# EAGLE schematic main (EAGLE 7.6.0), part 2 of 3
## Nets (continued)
U_DMA_9: IC37.15(D4)
U_DMA_10: IC38.15(D4)
U_DMA_11: IC40.15(D4)
U_DMA_12: IC41.15(D4)
U_DMA_13: IC71.15(D4)
U_DMA_14: IC20.15(D4)
U_DMA_15: IC172.15(D4)
U_FETCH_0: IC186.2(D2)
U_FETCH_1: IC160.2(D2)
U_FETCH_2: IC159.2(D2)
U_FETCH_3: IC142.2(D2)
U_FETCH_4: IC129.2(D2)
U_FETCH_5: IC73.2(D2)
U_FETCH_6: IC34.2(D2)
U_FETCH_7: IC35.2(D2)
U_FETCH_8: IC36.2(D2)
U_FETCH_9: IC37.2(D2)
U_FETCH_10: IC38.2(D2)
U_FETCH_11: IC40.2(D2)
U_FETCH_12: IC41.2(D2)
U_FETCH_13: IC71.2(D2)
U_FETCH_14: IC20.2(D2)
U_FETCH_15: IC172.2(D2)
U_FLAGS_REG_WRT: IC126.1(G)
U_INT_0: IC186.14(D5)
U_INT_1: IC160.14(D5)
U_INT_2: IC159.14(D5)
U_INT_3: IC142.14(D5)
U_INT_4: IC129.14(D5)
U_INT_5: IC73.14(D5)
U_INT_6: IC34.14(D5)
U_INT_7: IC35.14(D5)
U_INT_8: IC36.14(D5)
U_INT_9: IC37.14(D5)
U_INT_10: IC38.14(D5)
U_INT_11: IC40.14(D5)
U_INT_12: IC41.14(D5)
U_INT_13: IC71.14(D5)
U_INT_14: IC20.14(D5)
U_INT_15: IC172.14(D5)
U_OF: IC126.9(4Q) IC156.11(2C1)
U_OFFSET0: IC49.3(1B)
U_OFFSET1: IC49.6(2B)
U_OFFSET2: IC49.10(3B)
U_OFFSET3: IC49.13(4B)
U_OFFSET4: IC55.3(1B)
U_OFFSET5: IC55.6(2B)
U_OFFSET6: IC55.10(3B) IC55.13(4B) IC63.3(1B) IC63.6(2B) IC63.10(3B) IC63.13(4B) IC68.3(1B) IC68.6(2B) IC68.10(3B) IC68.13(4B)
U_SF: IC126.6(3Q) IC156.5(1C1)
U_TRAP_0: IC186.1(D3)
U_TRAP_1: IC160.1(D3)
U_TRAP_2: IC159.1(D3)
U_TRAP_3: IC142.1(D3)
U_TRAP_4: IC129.1(D3)
U_TRAP_5: IC73.1(D3)
U_TRAP_6: IC34.1(D3)
U_TRAP_7: IC35.1(D3)
U_TRAP_8: IC36.1(D3)
U_TRAP_9: IC37.1(D3)
U_TRAP_10: IC38.1(D3)
U_TRAP_11: IC40.1(D3)
U_TRAP_12: IC41.1(D3)
U_TRAP_13: IC71.1(D3)
U_TRAP_14: IC20.1(D3)
U_TRAP_15: IC172.1(D3)
U_ZF: IC46.1(A:I0) IC126.2(1Q) IC127.2(A:I1) IC155.5(1C1)
U_ZF_IN_SRC: IC121.1(!A!/B)
VAR_SPEED_CLK: SW1.4
VCC: IC8.2(A:D) IC8.4(A:PRE) IC39.2(A:D) IC39.4(A:PRE) IC49.2(1A) IC56.5(1C1) IC163.2(A:D) IC163.4(A:PRE) IC164.2(A:D) IC164.4(A:PRE) IC168.2(A:D) IC168.4(A:PRE) IC174.2(A:D) IC174.4(A:PRE) IC187.2(A:D) IC187.4(A:PRE) IC188.2(A:D) IC188.4(A:PRE) IC204.4(A:PRE) IC221.2(A:D) IC221.4(A:PRE) IC222.6(G1) IC413.1(A:CLR) R23.2 R24.2 R25.2 R26.2 RN7.9 RN7.10 RN7.11 RN7.12 RN7.13 RN7.14 RN7.15 RN7.16
WR: IC60.5(Q2) IC69.13(B:A2)
XBUS0: IC2.18(Y1) IC9.18(Y1) IC25.9(B:Y1) IC27.9(B:Y1) IC29.18(Y1) IC87.18(Y1) IC91.18(Y1) IC92.18(Y1) IC116.18(Y1) IC117.18(Y1) IC122.18(Y1) IC125.18(Y1) IC140.18(Y1) IC145.18(Y1) IC154.18(Y1) IC181.18(A:Y1) IC210.18(Y1) IC245.18(Y1)
XBUS1: IC2.17(Y2) IC9.17(Y2) IC25.7(B:Y2) IC27.7(B:Y2) IC29.17(Y2) IC87.17(Y2) IC116.17(Y2) IC117.17(Y2) IC122.17(Y2) IC125.17(Y2) IC145.17(Y2) IC154.17(Y2) IC181.16(A:Y2) IC245.17(Y2)
XBUS2: IC2.16(Y3) IC9.16(Y3) IC25.5(B:Y3) IC27.5(B:Y3) IC29.16(Y3) IC87.16(Y3) IC116.16(Y3) IC117.16(Y3) IC122.16(Y3) IC125.16(Y3) IC145.16(Y3) IC154.16(Y3) IC181.14(A:Y3) IC245.16(Y3)
XBUS3: IC2.15(Y4) IC9.15(Y4) IC25.3(B:Y4) IC27.3(B:Y4) IC29.15(Y4) IC87.15(Y4) IC116.15(Y4) IC117.15(Y4) IC122.15(Y4) IC125.15(Y4) IC145.15(Y4) IC154.15(Y4) IC181.12(A:Y4) IC245.15(Y4)
XBUS4: IC24.9(B:Y1) IC26.9(B:Y1) IC29.14(Y5) IC87.14(Y5) IC116.14(Y5) IC125.14(Y5) IC154.14(Y5) IC176.18(A:Y1) IC245.14(Y5)
XBUS5: IC24.7(B:Y2) IC26.7(B:Y2) IC29.13(Y6) IC87.13(Y6) IC116.13(Y6) IC125.13(Y6) IC154.13(Y6) IC176.16(A:Y2) IC245.13(Y6)
XBUS6: IC24.5(B:Y3) IC26.5(B:Y3) IC29.12(Y7) IC87.12(Y7) IC115.12(Y7) IC116.12(Y7) IC125.12(Y7) IC154.12(Y7) IC176.14(A:Y3) IC245.12(Y7)
XBUS7: IC2.11(Y8) IC3.11(Y8) IC9.11(Y8) IC24.3(B:Y4) IC26.3(B:Y4) IC29.11(Y8) IC80.4(B:I0) IC87.11(Y8) IC91.11(Y8) IC92.11(Y8) IC102.11(Y8) IC115.11(Y8) IC116.11(Y8) IC117.11(Y8) IC122.11(Y8) IC125.11(Y8) IC130.5(B:I1) IC140.11(Y8) IC145.11(Y8) IC146.11(Y8) IC154.11(Y8) IC176.12(A:Y4) IC210.11(Y8) IC245.11(Y8)
XBUS8: IC146.18(Y1)
XBUS9: IC146.17(Y2)
XBUS10: IC146.16(Y3)
XBUS11: IC146.15(Y4)
XBUS12: IC171.18(Y1) IC215.18(Y1)
XBUS13: IC171.11(Y8) IC215.11(Y8)
XBUS14: IC259.18(Y1) IC260.18(Y1)
XBUS15: IC259.11(Y8) IC260.11(Y8)
XBUS16: IC244.9(B:Y1)
XBUS17: IC244.3(B:Y4)
XBUS18: IC247.9(B:Y1)
XBUS19: IC247.3(B:Y4)
XBUS20: IC105.9(B:Y1) IC107.9(B:Y1)
XBUS21: IC105.7(B:Y2) IC107.7(B:Y2)
XBUS22: IC105.5(B:Y3) IC107.5(B:Y3)
XBUS23: IC105.3(B:Y4) IC107.3(B:Y4)
XBUS24: IC14.1(B0) RN2.1
XBUS25: IC14.22(B1) RN2.2
XBUS26: IC14.20(B2) RN2.3
XBUS27: IC14.18(B3) RN2.4
XBUS28: IC11.12(A:Y4) IC15.1(B0) RN2.5
XBUS29: IC11.14(A:Y3) IC15.22(B1) RN2.6
XBUS30: IC11.16(A:Y2) IC15.20(B2) RN2.7
XBUS31: IC11.18(A:Y1) IC15.18(B3) RN2.8
XBUS32: IC102.18(Y1)
XBUS33: IC102.17(Y2)
XBUS34: IC102.16(Y3)
XBUS35: IC102.15(Y4)
XBUS36: IC263.18(Y1) IC264.18(Y1)
XBUS37: IC263.11(Y8) IC264.11(Y8)
XBUS38: IC252.18(Y1) IC253.18(Y1)
XBUS39: IC252.11(Y8) IC253.11(Y8)
XBUS40: IC3.18(Y1)
XBUS41: IC3.17(Y2)
XBUS42: IC3.16(Y3)
XBUS43: IC3.15(Y4)
XBUS44: IC266.18(Y1) IC267.18(Y1)
XBUS45: IC266.11(Y8) IC267.11(Y8)
XBUS46: IC298.18(A:Y1)
XBUS47: IC298.16(A:Y2)
XBUS48: IC115.18(Y1)
XBUS49: IC115.17(Y2)
XBUS50: IC115.16(Y3)
XBUS51: IC115.15(Y4)
XBUS52: IC298.14(A:Y3)
XBUS53: IC298.12(A:Y4)
XBUS54: IC297.18(A:Y1)
XBUS55: IC297.16(A:Y2)
XBUS56: IC15.19(A3) RN3.1
XBUS57: IC15.21(A2) RN3.2
XBUS58: IC15.23(A1) RN3.3
XBUS59: IC15.2(A0) RN3.4
XBUS60: IC14.19(A3) RN3.5
XBUS61: IC14.21(A2) RN3.6
XBUS62: IC14.23(A1) RN3.7
XBUS63: IC14.2(A0) RN3.8
XBUS64: IC297.14(A:Y3)
XBUS65: IC297.12(A:Y4)
XBUS66: IC289.12(A:Y4)
XBUS67: IC289.14(A:Y3)
XBUS68: IC289.16(A:Y2)
XBUS69: IC289.18(A:Y1)
XBUS70: IC106.9(B:Y1) IC108.9(B:Y1)
XBUS71: IC106.7(B:Y2) IC108.7(B:Y2)
XBUS72: IC106.5(B:Y3) IC108.5(B:Y3)
XBUS73: IC106.3(B:Y4) IC108.3(B:Y4)
XBUS74: IC113.18(Y1) IC114.18(Y1)
XBUS75: IC113.17(Y2) IC114.17(Y2)
XBUS76: IC113.16(Y3) IC114.16(Y3)
XBUS77: IC113.15(Y4) IC114.15(Y4)
XBUS78: IC113.12(Y7) IC114.12(Y7)
XBUS79: IC113.11(Y8) IC114.11(Y8)
XBUS80: IC109.9(B:Y1) IC111.9(B:Y1)
XBUS81: IC109.7(B:Y2) IC111.7(B:Y2)
XBUS82: IC109.5(B:Y3) IC111.5(B:Y3)
XBUS83: IC109.3(B:Y4) IC111.3(B:Y4)
XBUS84: IC110.9(B:Y1) IC112.9(B:Y1)
XBUS85: IC110.7(B:Y2) IC112.7(B:Y2)
XBUS86: IC110.5(B:Y3) IC112.5(B:Y3)
XBUS87: IC110.3(B:Y4) IC112.3(B:Y4)
YBUS0: IC44.18(Y1) IC139.18(Y1) IC182.18(A:Y1)
YBUS1: IC44.17(Y2) IC139.17(Y2) IC182.16(A:Y2)
YBUS2: IC44.16(Y3) IC139.16(Y3) IC182.14(A:Y3)
YBUS3: IC44.15(Y4) IC139.15(Y4) IC182.12(A:Y4)
YBUS4: IC44.14(Y5) IC139.14(Y5) IC183.18(A:Y1)
YBUS5: IC44.13(Y6) IC139.13(Y6) IC183.16(A:Y2)
YBUS6: IC44.12(Y7) IC139.12(Y7) IC183.14(A:Y3)
YBUS7: IC44.11(Y8) IC130.4(B:I0) IC139.11(Y8) IC183.12(A:Y4)
YBUS8: IC299.18(A:Y1)
YBUS9: IC299.16(A:Y2)
YBUS10: IC299.14(A:Y3)
YBUS11: IC299.12(A:Y4)
YBUS12: IC300.18(A:Y1)
YBUS13: IC300.16(A:Y2)
YBUS14: IC300.14(A:Y3)
YBUS15: IC300.12(A:Y4)
YBUS16: IC16.18(Y1)
YBUS17: IC16.17(Y2)
YBUS18: IC16.16(Y3)
YBUS19: IC16.15(Y4)
YBUS20: IC16.14(Y5)
YBUS21: IC16.11(Y8)
ZBUFF1_0: IC98.3(1D) IC99.3(1D)
ZBUFF1_1: IC98.4(2D) IC99.4(2D)
ZBUFF1_2: IC98.7(3D) IC99.7(3D)
ZBUFF1_3: IC98.8(4D) IC99.8(4D)
ZBUFF1_4: IC98.13(5D) IC99.13(5D)
ZBUFF1_5: IC98.14(6D) IC99.14(6D)
ZBUFF1_6: IC98.17(7D) IC99.17(7D)
ZBUFF1_7: IC98.18(8D) IC99.18(8D)
ZBUFF1_8: IC173.3(1D) IC205.3(1D)
ZBUFF1_9: IC173.4(2D) IC205.4(2D)
ZBUFF1_10: IC173.7(3D) IC205.7(3D)
ZBUFF1_11: IC173.8(4D) IC205.8(4D)
ZBUFF1_12: IC173.13(5D) IC205.13(5D)
ZBUFF1_13: IC173.14(6D) IC205.14(6D)
ZBUFF1_14: IC173.17(7D) IC205.17(7D)
ZBUFF1_15: IC173.18(8D) IC205.18(8D)
ZBUFF1_16: IC165.3(1D) IC166.3(1D)
ZBUFF1_17: IC165.4(2D) IC166.4(2D)
ZBUFF1_18: IC165.7(3D) IC166.7(3D)
ZBUFF1_19: IC165.8(4D) IC166.8(4D)
ZBUFF1_20: IC165.13(5D) IC166.13(5D)
ZBUFF1_21: IC165.14(6D) IC166.14(6D)
ZBUFF1_22: IC165.17(7D) IC166.17(7D)
ZBUFF1_23: IC165.18(8D) IC166.18(8D)
ZBUFF1_24: IC217.3(1D) IC246.3(1D)
ZBUFF1_25: IC217.4(2D) IC246.4(2D)
ZBUFF1_26: IC217.7(3D) IC246.7(3D)
ZBUFF1_27: IC217.8(4D) IC246.8(4D)
ZBUFF1_28: IC217.13(5D) IC246.13(5D)
ZBUFF1_29: IC217.14(6D) IC246.14(6D)
ZBUFF1_30: IC217.17(7D) IC246.17(7D)
ZBUFF1_31: IC217.18(8D) IC246.18(8D)
ZBUFF1_32: IC261.3(1D) IC262.3(1D)
ZBUFF1_33: IC261.4(2D) IC262.4(2D)
ZBUFF1_34: IC261.7(3D) IC262.7(3D)
ZBUFF1_35: IC261.8(4D) IC262.8(4D)
ZBUFF1_36: IC261.13(5D) IC262.13(5D)
ZBUFF1_37: IC261.14(6D) IC262.14(6D)
ZBUFF1_38: IC261.17(7D) IC262.17(7D)
ZBUFF1_39: IC261.18(8D) IC262.18(8D)
ZBUFF1_40: IC202.3(1D) IC251.3(1D)
ZBUFF1_41: IC202.4(2D) IC251.4(2D)
ZBUFF1_42: IC202.7(3D) IC251.7(3D)
ZBUFF1_43: IC202.8(4D) IC251.8(4D)
ZBUFF1_44: IC202.13(5D) IC251.13(5D)
ZBUFF1_45: IC202.14(6D) IC251.14(6D)
ZBUFF1_46: IC202.17(7D) IC251.17(7D)
ZBUFF1_47: IC202.18(8D) IC251.18(8D)
ZBUFF1_48: IC254.3(1D) IC265.3(1D)
ZBUFF1_49: IC254.4(2D) IC265.4(2D)
ZBUFF1_50: IC254.7(3D) IC265.7(3D)
ZBUFF1_51: IC254.8(4D) IC265.8(4D)
ZBUFF1_52: IC254.13(5D) IC265.13(5D)
ZBUFF1_53: IC254.14(6D) IC265.14(6D)
ZBUFF1_54: IC254.17(7D) IC265.17(7D)
ZBUFF1_55: IC254.18(8D) IC265.18(8D)
ZBUFF1_56: IC4.3(1D) IC5.3(1D)
ZBUFF1_57: IC4.4(2D) IC5.4(2D)
ZBUFF1_58: IC4.7(3D) IC5.7(3D)
ZBUFF1_59: IC4.8(4D) IC5.8(4D)
ZBUFF1_60: IC4.13(5D) IC5.13(5D)
ZBUFF1_61: IC4.14(6D) IC5.14(6D)
ZBUFF1_62: IC4.17(7D) IC5.17(7D)
ZBUFF1_63: IC4.18(8D) IC5.18(8D)
ZBUFF2_0: IC1.3(1D) IC23.14(4A) IC100.3(1D) IC101.3(1D)
ZBUFF2_1: IC1.4(2D) IC23.11(3A) IC100.4(2D) IC101.4(2D)
ZBUFF2_2: IC1.7(3D) IC23.5(2A) IC100.7(3D) IC101.7(3D)
ZBUFF2_3: IC1.8(4D) IC23.2(1A) IC100.8(4D) IC101.8(4D)
ZBUFF2_4: IC1.13(5D) IC22.14(4A) IC100.13(5D) IC101.13(5D)
ZBUFF2_5: IC1.14(6D) IC22.11(3A) IC100.14(6D) IC101.14(6D)
ZBUFF2_6: IC1.17(7D) IC22.5(2A) IC100.17(7D) IC101.17(7D)
ZBUFF2_7: IC22.2(1A) IC100.18(8D) IC101.18(8D)
ZBUFF2_16: IC123.3(1D)
ZBUFF2_17: IC123.4(2D)
ZBUFF2_18: IC123.7(3D)
ZBUFF2_19: IC123.8(4D)
ZBUFF2_20: IC123.13(5D)
ZBUFF2_21: IC123.14(6D)
ZBUFF2_22: IC123.17(7D)
ZBUFF2_23: IC153.3(1D)
ZBUFF2_24: IC153.4(2D)
ZBUFF2_25: IC153.7(3D)
ZBUFF2_26: IC153.8(4D)
ZBUFF2_27: IC153.13(5D)
ZBUFF2_28: IC153.14(6D)
ZBUFF2_29: IC153.17(7D)
ZBUFF2_30: IC153.18(8D)
ZBUFF2_31: IC185.3(1D)
ZBUFF2_32: IC185.4(2D)
ZBUFF2_33: IC185.7(3D)
ZBUFF2_34: IC185.8(4D)
ZBUFF2_35: IC185.13(5D)
ZBUFF2_36: IC185.14(6D)
ZBUFF2_37: IC185.17(7D)
ZBUFF2_38: IC185.18(8D)
ZBUS0: IC7.3(1D) IC54.3(1D) IC95.6(B1) IC96.3(1B) IC103.3(1B) IC144.14(D1) IC175.4(B:I0) IC184.3(1D) IC189.3(1D) IC197.1(A:I0) IC216.3(1D) IC241.3(1C3) IC544.3(1D) RN1.1 RN5.1 RN7.8
ZBUS1: IC54.4(2D) IC95.2(B2) IC96.6(2B) IC103.6(2B) IC144.13(D2) IC175.5(B:I1) IC184.4(2D) IC197.2(A:I1) IC216.4(2D) IC243.3(1C3) IC544.4(2D) RN1.2 RN5.2 RN7.7
ZBUS2: IC54.7(3D) IC95.15(B3) IC96.10(3B) IC103.10(3B) IC144.12(D3) IC177.5(B:I1) IC184.7(3D) IC197.3(A:I2) IC216.7(3D) IC255.3(1C3) IC544.7(3D) RN1.3 RN5.3 RN7.6
ZBUS3: IC54.8(4D) IC95.11(B4) IC96.13(4B) IC103.13(4B) IC144.11(D4) IC184.8(4D) IC192.5(B:I1) IC197.12(A:I3) IC216.8(4D) IC256.3(1C3) IC544.8(4D) RN1.4 RN5.4 RN7.5
ZBUS4: IC54.13(5D) IC97.3(1B) IC104.3(1B) IC119.6(B1) IC128.14(D1) IC184.13(5D) IC193.5(B:I1) IC197.13(A:I4) IC208.3(1C3) IC216.13(5D) IC544.13(5D) RN1.5 RN5.5 RN7.4
ZBUS5: IC54.14(6D) IC97.6(2B) IC104.6(2B) IC119.2(B2) IC128.13(D2) IC184.14(6D) IC194.5(B:I1) IC199.2(A:I1) IC216.14(6D) IC544.14(6D) RN1.6 RN5.6 RN7.3
ZBUS6: IC54.17(7D) IC97.10(3B) IC104.10(3B) IC119.15(B3) IC128.12(D3) IC184.17(7D) IC199.3(A:I2) IC200.5(B:I1) IC216.17(7D) IC544.17(7D) RN1.7 RN5.7 RN7.2
ZBUS7: IC7.18(8D) IC54.18(8D) IC80.5(B:I1) IC97.13(4B) IC104.13(4B) IC119.11(B4) IC124.2(B2) IC124.6(B1) IC124.11(B4) IC124.15(B3) IC128.11(D4) IC148.2(B2) IC148.6(B1) IC148.11(B4) IC148.15(B3) IC184.18(8D) IC189.18(8D) IC199.12(A:I3) IC209.5(B:I1) IC216.18(8D) IC255.5(1C1) IC544.18(8D) RN1.8 RN5.8 RN7.1
ZBUS8: IC89.2(1A) IC90.2(1A)
ZBUS9: IC89.5(2A) IC90.5(2A)
ZBUS10: IC89.11(3A) IC90.11(3A)
ZBUS11: IC89.14(4A) IC90.14(4A)
ZBUS12: IC86.2(1A) IC88.2(1A)
ZBUS13: IC86.5(2A) IC88.5(2A)
ZBUS14: IC86.11(3A) IC88.11(3A)
ZBUS15: IC86.14(4A) IC88.14(4A)
ZBUS16: IC248.14(D1)
ZBUS17: IC248.13(D2)
ZBUS18: IC248.12(D3)
ZBUS19: IC248.11(D4)
ZBUS20: IC249.14(D1)
ZBUS21: IC249.13(D2)
ZBUS22: IC249.12(D3)
ZBUS23: IC249.11(D4)
ZF: IC120.2(A:I1) IC122.2(A1) IC155.6(1C0) IC227.2(Q1) IC241.6(1C0)
ZF_FROM_ALU: IC46.2(A:I1) IC120.1(A:I0) IC121.2(1A) IC127.1(A:I0) IC155.4(1C2) IC199.5(A:O) IC241.5(1C1)
ZF_IN_SRC_0: IC241.14(A)
ZF_IN_SRC_1: IC241.2(B)
~CLK: IC32.11(CLK) IC33.11(CLK)
~RST: IC32.1(CLR) IC33.1(CLR) IC42.1(A:I0) IC162.1(CLR) IC195.1(A:I0) IC204.1(A:CLR) IC207.2(A:I1) IC218.1(A:I0) IC219.1(A:I0) IC220.2(A:I1) IC223.2(A:I1) IC224.2(A:I1) IC225.2(A:I1) IC227.1(CLR) IC413.4(A:PRE) IC414.4(B:O)
Unconnected: IC1.11(CLK) IC1.18(8D) IC2.12(Y7) IC2.13(Y6) IC2.14(Y5) IC3.12(Y7) IC3.13(Y6) IC3.14(Y5) IC4.11(CLK) IC5.11(CLK) IC6.11(CLK) IC7.4(2D) IC7.7(3D) IC7.8(4D) IC7.13(5D) IC7.14(6D) IC7.17(7D) IC8.6(A:!Q) IC8.8(B:!Q) IC8.9(B:Q) IC8.10(B:PRE) IC8.11(B:CLK) IC8.12(B:D) IC8.13(B:CLR) IC9.12(Y7) IC9.13(Y6) IC9.14(Y5) IC10.3(B:Y4) IC10.5(B:Y3) IC10.7(B:Y2) IC10.9(B:Y1) IC10.11(B:A1) IC10.13(B:A2) IC10.15(B:A3) IC10.17(B:A4) IC10.19(B:G) IC11.3(B:Y4) IC11.5(B:Y3) IC11.7(B:Y2) IC11.9(B:Y1) IC11.11(B:A1) IC11.13(B:A2) IC11.15(B:A3) IC11.17(B:A4) IC11.19(B:G) IC12.3(B:Y4) IC12.5(B:Y3) IC12.7(B:Y2) IC12.9(B:Y1) IC12.11(B:A1) IC12.13(B:A2) IC12.15(B:A3) IC12.17(B:A4) IC12.19(B:G) IC13.3(B:Y4) IC13.5(B:Y3) IC13.7(B:Y2) IC13.9(B:Y1) IC13.11(B:A1) IC13.13(B:A2) IC13.15(B:A3) IC13.17(B:A4) IC13.19(B:G) IC14.14(A=B) IC14.15(P) IC14.17(G) IC15.14(A=B) IC15.15(P) IC15.17(G) IC16.2(A1) IC16.3(A2) IC16.4(A3) IC16.5(A4) IC16.6(A5) IC16.7(A6) IC16.8(A7) IC16.9(A8) IC16.12(Y7) IC16.13(Y6) IC17.11(CLK) IC18.1(A:I0) IC18.2(A:I1) IC18.3(A:O) IC18.8(C:O) IC18.9(C:I0) IC18.10(C:I1) IC18.11(D:O) IC18.12(D:I0) IC18.13(D:I1) IC19.11(CLK) IC20.6(W) IC20.7(G) IC20.9(C) IC20.10(B) IC20.11(A) IC20.12(D7) IC20.13(D6) IC21.11(CLK) IC24.1(A:G) IC24.2(A:A1) IC24.4(A:A2) IC24.6(A:A3) IC24.8(A:A4) IC24.12(A:Y4) IC24.14(A:Y3) IC24.16(A:Y2) IC24.18(A:Y1) IC25.1(A:G) IC25.2(A:A1) IC25.4(A:A2) IC25.6(A:A3) IC25.8(A:A4) IC25.12(A:Y4) IC25.14(A:Y3) IC25.16(A:Y2) IC25.18(A:Y1) IC26.1(A:G) IC26.2(A:A1) IC26.4(A:A2) IC26.6(A:A3) IC26.8(A:A4) IC26.12(A:Y4) IC26.14(A:Y3) IC26.16(A:Y2) IC26.18(A:Y1) IC27.1(A:G) IC27.2(A:A1) IC27.4(A:A2) IC27.6(A:A3) IC27.8(A:A4) IC27.12(A:Y4) IC27.14(A:Y3) IC27.16(A:Y2) IC27.18(A:Y1) IC28.6(A5) IC28.7(A6) IC28.8(A7) IC28.9(A8) IC28.11(Y8) IC28.12(Y7) IC28.13(Y6) IC28.14(Y5) IC29.7(A6) IC29.8(A7) IC29.9(A8) IC30.3(B:Y4) IC30.5(B:Y3) IC30.7(B:Y2) IC30.9(B:Y1) IC30.11(B:A1) IC30.13(B:A2) IC30.15(B:A3) IC30.17(B:A4) IC30.19(B:G) IC31.3(B:Y4) IC31.5(B:Y3) IC31.7(B:Y2) IC31.9(B:Y1) IC31.11(B:A1) IC31.13(B:A2) IC31.15(B:A3) IC31.17(B:A4) IC31.19(B:G) IC34.6(W) IC34.7(G) IC34.9(C) IC34.10(B) IC34.11(A) IC34.12(D7) IC34.13(D6) IC35.6(W) IC35.7(G) IC35.9(C) IC35.10(B) IC35.11(A) IC35.12(D7) IC35.13(D6) IC36.6(W) IC36.7(G) IC36.9(C) IC36.10(B) IC36.11(A) IC36.12(D7) IC36.13(D6) IC37.6(W) IC37.7(G) IC37.9(C) IC37.10(B) IC37.11(A) IC37.12(D7) IC37.13(D6) IC38.6(W) IC38.7(G) IC38.9(C) IC38.10(B) IC38.11(A) IC38.12(D7) IC38.13(D6) IC39.6(A:!Q) IC39.8(B:!Q) IC39.9(B:Q) IC39.10(B:PRE) IC39.11(B:CLK) IC39.12(B:D) IC39.13(B:CLR) IC40.6(W) IC40.7(G) IC40.9(C) IC40.10(B) IC40.11(A) IC40.12(D7) IC40.13(D6) IC41.6(W) IC41.7(G) IC41.9(C) IC41.10(B) IC41.11(A) IC41.12(D7) IC41.13(D6) IC42.4(B:I0) IC42.5(B:I1) IC42.6(B:O) IC42.8(C:O) IC42.9(C:I0) IC42.10(C:I1) IC42.11(D:O) IC42.12(D:I0) IC42.13(D:I1) IC43.1(A:I) IC43.2(A:O) IC43.5(C:I) IC43.6(C:O) IC43.8(D:O) IC43.9(D:I) IC43.10(E:O) IC43.11(E:I) IC43.12(F:O) IC43.13(F:I) IC45.4(B:I0) IC45.5(B:I1) IC45.6(B:O) IC45.8(C:O) IC45.9(C:I0) IC45.10(C:I1) IC45.11(D:O) IC45.12(D:I0) IC45.13(D:I1) IC46.4(B:I0) IC46.5(B:I1) IC46.6(B:O) IC46.8(C:O) IC46.9(C:I0) IC46.10(C:I1) IC46.11(D:O) IC46.12(D:I0) IC46.13(D:I1) IC47.4(B:I0) IC47.5(B:I1) IC47.6(B:O) IC47.8(C:O) IC47.9(C:I0) IC47.10(C:I1) IC47.11(D:O) IC47.12(D:I0) IC47.13(D:I1) IC48.11(CLK) IC50.1(S2) IC50.10(S4) IC50.13(S3) IC51.1(S2) IC51.4(S1) IC51.10(S4) IC51.13(S3) IC52.1(S2) IC52.4(S1) IC52.10(S4) IC52.13(S3) IC53.4(S1) IC53.9(C4) IC53.10(S4) IC53.13(S3) IC54.11(CLK) IC56.9(2Y) IC56.10(2C0) IC56.11(2C1) IC56.12(2C2) IC56.13(2C3) IC57.3(B:I) IC57.4(B:O) IC57.5(C:I) IC57.6(C:O) IC57.8(D:O) IC57.9(D:I) IC57.10(E:O) IC57.11(E:I) IC57.12(F:O) IC57.13(F:I) IC58.4(B:I0) IC58.5(B:I1) IC58.6(B:O) IC58.8(C:O) IC58.9(C:I0) IC58.10(C:I1) IC58.11(D:O) IC58.12(D:I0) IC58.13(D:I1) IC59.3(B:I) IC59.4(B:O) IC59.5(C:I) IC59.6(C:O) IC59.8(D:O) IC59.9(D:I) IC59.10(E:O) IC59.11(E:I) IC59.12(F:O) IC59.13(F:I) IC60.1(CLR) IC60.9(Q4) IC60.12(Q5) IC60.15(Q6) IC60.16(Q7) IC60.19(Q8) IC61.1(CLR) IC61.2(Q1) IC61.5(Q2) IC61.6(Q3) IC61.9(Q4) IC61.12(Q5) IC61.15(Q6) IC61.16(Q7) IC61.19(Q8) IC62.1(CLR) IC62.2(Q1) IC62.5(Q2) IC62.6(Q3) IC62.9(Q4) IC62.12(Q5) IC62.15(Q6) IC62.16(Q7) IC62.19(Q8) IC64.3(B:I0) IC64.4(B:I1) IC64.5(B:I2) IC64.6(B:O) IC64.8(C:O) IC64.9(C:I0) IC64.10(C:I1) IC64.11(C:I2) IC65.4(B:O) IC65.5(B:I0) IC65.6(B:I1) IC65.8(C:I0) IC65.9(C:I1) IC65.10(C:O) IC65.11(D:I0) IC65.12(D:I1) IC65.13(D:O) IC66.4(B:O) IC66.5(B:I0) IC66.6(B:I1) IC66.8(C:I0) IC66.9(C:I1) IC66.10(C:O) IC66.11(D:I0) IC66.12(D:I1) IC66.13(D:O) IC69.1(A:G) IC69.2(A:A1) IC69.3(B:Y4) IC69.4(A:A2) IC69.6(A:A3) IC69.8(A:A4) IC69.12(A:Y4) IC69.14(A:Y3) IC69.16(A:Y2) IC69.18(A:Y1) IC70.6(W) IC71.6(W) IC71.7(G) IC71.9(C) IC71.10(B) IC71.11(A) IC71.12(D7) IC71.13(D6) IC72.1(A:I0) IC72.2(A:I1) IC72.3(A:O) IC72.8(C:O) IC72.9(C:I0) IC72.10(C:I1) IC72.11(D:O) IC72.12(D:I0) IC72.13(D:I1) IC73.6(W) IC73.7(G) IC73.9(C) IC73.10(B) IC73.11(A) IC73.12(D7) IC73.13(D6) IC74.1(A:I0) IC74.2(A:I1) IC74.3(A:O) IC74.8(C:O) IC74.9(C:I0) IC74.10(C:I1) IC74.11(D:O) IC74.12(D:I0) IC74.13(D:I1) IC75.2(Q1) IC75.5(Q2) IC75.6(Q3) IC75.9(Q4) IC75.12(Q5) IC75.15(Q6) IC75.16(Q7) IC75.19(Q8) IC76.2(Q1) IC77.2(Q1) IC78.2(Q1) IC78.5(Q2) IC78.6(Q3) IC78.9(Q4) IC78.12(Q5) IC78.15(Q6) IC78.16(Q7) IC78.19(Q8) IC79.2(Q1) IC79.5(Q2) IC79.6(Q3) IC79.9(Q4) IC79.12(Q5) IC79.15(Q6) IC79.16(Q7) IC79.19(Q8) IC80.1(A:I0) IC80.2(A:I1) IC80.3(A:O) IC80.8(C:O) IC80.9(C:I0) IC80.10(C:I1) IC80.11(D:O) IC80.12(D:I0) IC80.13(D:I1) IC81.1(A:I0) IC81.2(A:I1) IC81.3(A:O) IC81.8(C:O) IC81.9(C:I0) IC81.10(C:I1) IC81.11(D:O) IC81.12(D:I0) IC81.13(D:I1) IC82.1(A:I0) IC82.2(A:I1) IC82.3(A:O) IC82.4(B:I0) IC82.5(B:I1) IC82.6(B:O) IC82.11(D:O) IC82.12(D:I0) IC82.13(D:I1) IC83.1(A:I) IC83.2(A:O) IC83.5(C:I) IC83.6(C:O) IC83.8(D:O) IC83.9(D:I) IC83.10(E:O) IC83.11(E:I) IC83.12(F:O) IC83.13(F:I) IC84.1(A:I) IC84.2(A:O) IC84.5(C:I) IC84.6(C:O) IC84.8(D:O) IC84.9(D:I) IC84.10(E:O) IC84.11(E:I) IC84.12(F:O) IC84.13(F:I) IC85.3(B:I0) IC85.4(B:I1) IC85.5(B:I2) IC85.6(B:O) IC85.8(C:O) IC85.9(C:I0) IC85.10(C:I1) IC85.11(C:I2) IC87.7(A6) IC87.8(A7) IC87.9(A8) IC91.12(Y7) IC91.13(Y6) IC91.14(Y5) IC91.15(Y4) IC91.16(Y3) IC91.17(Y2) IC92.12(Y7) IC92.13(Y6) IC92.14(Y5) IC92.15(Y4) IC92.16(Y3) IC92.17(Y2) IC93.3(B:I0) IC93.4(B:I1) IC93.5(B:I2) IC93.6(B:O) IC93.8(C:O) IC93.9(C:I0) IC93.10(C:I1) IC93.11(C:I2) IC94.1(A:I) IC94.2(A:O) IC94.5(C:I) IC94.6(C:O) IC94.8(D:O) IC94.9(D:I) IC94.10(E:O) IC94.11(E:I) IC94.12(F:O) IC94.13(F:I) IC96.15(G) IC97.15(G) IC98.11(CLK) IC99.11(CLK) IC100.11(CLK) IC101.11(CLK) IC102.12(Y7) IC102.13(Y6) IC102.14(Y5) IC103.15(G) IC104.15(G) IC105.1(A:G) IC105.2(A:A1) IC105.4(A:A2) IC105.6(A:A3) IC105.8(A:A4) IC105.12(A:Y4) IC105.14(A:Y3) IC105.16(A:Y2) IC105.18(A:Y1) IC106.1(A:G) IC106.2(A:A1) IC106.4(A:A2) IC106.6(A:A3) IC106.8(A:A4) IC106.12(A:Y4) IC106.14(A:Y3) IC106.16(A:Y2) IC106.18(A:Y1) IC107.1(A:G) IC107.2(A:A1) IC107.4(A:A2) IC107.6(A:A3) IC107.8(A:A4) IC107.12(A:Y4) IC107.14(A:Y3) IC107.16(A:Y2) IC107.18(A:Y1) IC108.1(A:G) IC108.2(A:A1) IC108.4(A:A2) IC108.6(A:A3) IC108.8(A:A4) IC108.12(A:Y4) IC108.14(A:Y3) IC108.16(A:Y2) IC108.18(A:Y1) IC109.1(A:G) IC109.2(A:A1) IC109.4(A:A2) IC109.6(A:A3) IC109.8(A:A4) IC109.12(A:Y4) IC109.14(A:Y3) IC109.16(A:Y2) IC109.18(A:Y1) IC110.1(A:G) IC110.2(A:A1) IC110.4(A:A2) IC110.6(A:A3) IC110.8(A:A4) IC110.12(A:Y4) IC110.14(A:Y3) IC110.16(A:Y2) IC110.18(A:Y1) IC111.1(A:G) IC111.2(A:A1) IC111.4(A:A2) IC111.6(A:A3) IC111.8(A:A4) IC111.12(A:Y4) IC111.14(A:Y3) IC111.16(A:Y2) IC111.18(A:Y1) IC112.1(A:G) IC112.2(A:A1) IC112.4(A:A2) IC112.6(A:A3) IC112.8(A:A4) IC112.12(A:Y4) IC112.14(A:Y3) IC112.16(A:Y2) IC112.18(A:Y1) IC113.13(Y6) IC113.14(Y5) IC113.19(G2) IC114.13(Y6) IC114.14(Y5) IC114.19(G2) IC115.13(Y6) IC115.14(Y5) IC117.12(Y7) IC117.13(Y6) IC117.14(Y5) IC118.11(CLK) IC118.12(5Q) IC118.15(6Q) IC118.16(7Q) IC118.19(8Q) IC120.4(B:I0) IC120.5(B:I1) IC120.6(B:O) IC120.8(C:O) IC120.9(C:I0) IC120.10(C:I1) IC120.11(D:O) IC120.12(D:I0) IC120.13(D:I1) IC121.5(2A) IC121.6(2B) IC121.7(2Y) IC121.9(3Y) IC121.10(3B) IC121.11(3A) IC121.12(4Y) IC121.13(4B) IC121.14(4A) IC122.12(Y7) IC122.13(Y6) IC122.14(Y5) IC123.11(CLK) IC123.18(8D) IC126.11(CLK) IC126.12(5Q) IC126.13(5D) IC126.14(6D) IC126.15(6Q) IC126.16(7Q) IC126.17(7D) IC126.18(8D) IC126.19(8Q) IC127.4(B:I0) IC127.5(B:I1) IC127.6(B:O) IC127.8(C:O) IC127.9(C:I0) IC127.10(C:I1) IC127.11(D:O) IC127.12(D:I0) IC127.13(D:I1) IC129.6(W) IC129.7(G) IC129.9(C) IC129.10(B) IC129.11(A) IC129.12(D7) IC129.13(D6) IC130.1(A:I0) IC130.2(A:I1) IC130.3(A:O) IC130.8(C:O) IC130.9(C:I0) IC130.10(C:I1) IC130.11(D:O) IC130.12(D:I0) IC130.13(D:I1) IC131.4(B:O) IC131.5(B:I0) IC131.6(B:I1) IC131.8(C:I0) IC131.9(C:I1) IC131.10(C:O) IC131.11(D:I0) IC131.12(D:I1) IC131.13(D:O) IC132.3(B:I0) IC132.4(B:I1) IC132.5(B:I2) IC132.6(B:O) IC132.8(C:O) IC132.9(C:I0) IC132.10(C:I1) IC132.11(C:I2) IC133.3(A:O) IC133.4(B:I0) IC133.5(B:I1) IC133.6(B:O) IC133.8(C:O) IC133.9(C:I0) IC133.10(C:I1) IC133.11(D:O) IC133.12(D:I0) IC133.13(D:I1) IC134.2(Q1) IC134.5(Q2) IC134.6(Q3) IC134.9(Q4) IC134.12(Q5) IC134.15(Q6) IC134.16(Q7) IC134.19(Q8) IC135.2(Q1) IC135.5(Q2) IC135.6(Q3) IC135.9(Q4) IC135.12(Q5) IC135.15(Q6) IC135.16(Q7) IC135.19(Q8) IC136.2(Q1) IC136.5(Q2) IC136.6(Q3) IC136.9(Q4) IC136.12(Q5) IC136.15(Q6) IC136.16(Q7) IC136.19(Q8) IC137.2(Q1) IC137.5(Q2) IC137.6(Q3) IC137.9(Q4) IC137.12(Q5) IC137.15(Q6) IC137.16(Q7) IC137.19(Q8) IC138.3(B:I0) IC138.4(B:I1) IC138.5(B:I2) IC138.6(B:O) IC138.8(C:O) IC138.9(C:I0) IC138.10(C:I1) IC138.11(C:I2) IC140.12(Y7) IC140.13(Y6) IC140.14(Y5) IC140.15(Y4) IC140.16(Y3) IC140.17(Y2) IC142.6(W) IC142.7(G) IC142.9(C) IC142.10(B) IC142.11(A) IC142.12(D7) IC142.13(D6) IC143.4(B:I0) IC143.5(B:I1) IC143.6(B:O) IC143.8(C:O) IC143.9(C:I0) IC143.10(C:I1) IC143.11(D:O) IC143.12(D:I0) IC143.13(D:I1) IC145.12(Y7) IC145.13(Y6) IC145.14(Y5) IC146.12(Y7) IC146.13(Y6) IC146.14(Y5) IC147.4(B:I0) IC147.5(B:I1) IC147.6(B:O) IC147.8(C:O) IC147.9(C:I0) IC147.10(C:I1) IC147.11(D:O) IC147.12(D:I0) IC147.13(D:I1) IC148.9(C4) IC149.1(A:I) IC149.2(A:O) IC149.5(C:I) IC149.6(C:O) IC149.8(D:O) IC149.9(D:I) IC149.10(E:O) IC149.11(E:I) IC149.12(F:O) IC149.13(F:I) IC150.3(B:I0) IC150.4(B:I1) IC150.5(B:I2) IC150.6(B:O) IC150.8(C:O) IC150.9(C:I0) IC150.10(C:I1) IC150.11(C:I2) IC151.3(B:I0) IC151.4(B:I1) IC151.5(B:I2) IC151.6(B:O) IC151.8(C:O) IC151.9(C:I0) IC151.10(C:I1) IC151.11(C:I2) IC152.1(A:I0) IC152.2(A:I1) IC152.3(A:O) IC152.4(B:I0) IC152.5(B:I1) IC152.6(B:O) IC152.11(D:O) IC152.12(D:I0) IC152.13(D:I1) IC153.11(CLK) IC155.13(2C3) IC156.3(1C3) IC156.13(2C3) IC157.3(B:I0) IC157.4(B:I1) IC157.5(B:I2) IC157.6(B:O) IC157.8(C:O) IC157.9(C:I0) IC157.10(C:I1) IC157.11(C:I2) IC158.3(B:I0) IC158.4(B:I1) IC158.5(B:I2) IC158.6(B:O) IC158.8(C:O) IC158.9(C:I0) IC158.10(C:I1) IC158.11(C:I2) IC159.6(W) IC159.7(G) IC159.9(C) IC159.10(B) IC159.11(A) IC159.12(D7) IC159.13(D6) IC160.6(W) IC160.7(G) IC160.9(C) IC160.10(B) IC160.11(A) IC160.12(D7) IC160.13(D6) IC161.15(G) IC163.6(A:!Q) IC163.8(B:!Q) IC163.9(B:Q) IC163.10(B:PRE) IC163.11(B:CLK) IC163.12(B:D) IC163.13(B:CLR) IC164.6(A:!Q) IC164.8(B:!Q) IC164.9(B:Q) IC164.10(B:PRE) IC164.11(B:CLK) IC164.12(B:D) IC164.13(B:CLR) IC165.11(CLK) IC166.11(CLK) IC167.5(2A) IC167.6(2B) IC167.7(2Y) IC167.9(3Y) IC167.10(3B) IC167.11(3A) IC167.12(4Y) IC167.13(4B) IC167.14(4A) IC168.6(A:!Q) IC168.8(B:!Q) IC168.9(B:Q) IC168.10(B:PRE) IC168.11(B:CLK) IC168.12(B:D) IC168.13(B:CLR) IC169.11(CLK) IC170.1(A:I0) IC170.2(A:I1) IC170.3(A:O) IC170.8(C:O) IC170.9(C:I0) IC170.10(C:I1) IC170.11(D:O) IC170.12(D:I0) IC170.13(D:I1) IC171.12(Y7) IC171.13(Y6) IC171.14(Y5) IC171.15(Y4) IC171.16(Y3) IC171.17(Y2) IC172.6(W) IC172.7(G) IC172.9(C) IC172.10(B) IC172.11(A) IC172.12(D7) IC172.13(D6) IC173.11(CLK) IC174.6(A:!Q) IC174.8(B:!Q) IC174.9(B:Q) IC174.10(B:PRE) IC174.11(B:CLK) IC174.12(B:D) IC174.13(B:CLR) IC175.1(A:I0) IC175.2(A:I1) IC175.3(A:O) IC175.8(C:O) IC175.9(C:I0) IC175.10(C:I1) IC175.11(D:O) IC175.12(D:I0) IC175.13(D:I1) IC176.3(B:Y4) IC176.5(B:Y3) IC176.7(B:Y2) IC176.9(B:Y1) IC176.11(B:A1) IC176.13(B:A2) IC176.15(B:A3) IC176.17(B:A4) IC176.19(B:G) IC177.1(A:I0) IC177.2(A:I1) IC177.3(A:O) IC177.8(C:O) IC177.9(C:I0) IC177.10(C:I1) IC177.11(D:O) IC177.12(D:I0) IC177.13(D:I1) IC178.3(B:Y4) IC178.5(B:Y3) IC178.7(B:Y2) IC178.9(B:Y1) IC178.11(B:A1) IC178.13(B:A2) IC178.15(B:A3) IC178.17(B:A4) IC178.19(B:G) IC179.3(B:Y4) IC179.5(B:Y3) IC179.7(B:Y2) IC179.9(B:Y1) IC179.11(B:A1) IC179.13(B:A2) IC179.15(B:A3) IC179.17(B:A4) IC179.19(B:G) IC180.11(CLK) IC181.3(B:Y4) IC181.5(B:Y3) IC181.7(B:Y2) IC181.9(B:Y1) IC181.11(B:A1) IC181.13(B:A2) IC181.15(B:A3) IC181.17(B:A4) IC181.19(B:G) IC182.3(B:Y4) IC182.5(B:Y3) IC182.7(B:Y2) IC182.9(B:Y1) IC182.11(B:A1) IC182.13(B:A2) IC182.15(B:A3) IC182.17(B:A4) IC182.19(B:G) IC183.3(B:Y4) IC183.5(B:Y3) IC183.7(B:Y2) IC183.9(B:Y1) IC183.11(B:A1) IC183.13(B:A2) IC183.15(B:A3) IC183.17(B:A4) IC183.19(B:G) IC184.11(CLK) IC185.11(CLK) IC186.6(W) IC186.7(G) IC186.9(C) IC186.10(B) IC186.11(A) IC186.12(D7) IC186.13(D6) IC187.6(A:!Q) IC187.8(B:!Q) IC187.9(B:Q) IC187.10(B:PRE) IC187.11(B:CLK) IC187.12(B:D) IC187.13(B:CLR) IC188.6(A:!Q) IC188.8(B:!Q) IC188.9(B:Q) IC188.10(B:PRE) IC188.11(B:CLK) IC188.12(B:D) IC188.13(B:CLR) IC189.4(2D) IC189.7(3D) IC189.8(4D) IC189.13(5D) IC189.14(6D) IC189.17(7D) IC190.1(A:I0) IC190.2(A:I1) IC190.3(A:O) IC190.4(B:I0) IC190.5(B:I1) IC190.6(B:O) IC190.11(D:O) IC190.12(D:I0) IC190.13(D:I1) IC191.3(B:I0) IC191.4(B:I1) IC191.5(B:I2) IC191.6(B:O) IC191.8(C:O) IC191.9(C:I0) IC191.10(C:I1) IC191.11(C:I2) IC192.1(A:I0) IC192.2(A:I1) IC192.3(A:O) IC192.8(C:O) IC192.9(C:I0) IC192.10(C:I1) IC192.11(D:O) IC192.12(D:I0) IC192.13(D:I1) IC193.1(A:I0) IC193.2(A:I1) IC193.3(A:O) IC193.8(C:O) IC193.9(C:I0) IC193.10(C:I1) IC193.11(D:O) IC193.12(D:I0) IC193.13(D:I1) IC194.1(A:I0) IC194.2(A:I1) IC194.3(A:O) IC194.8(C:O) IC194.9(C:I0) IC194.10(C:I1) IC194.11(D:O) IC194.12(D:I0) IC194.13(D:I1) IC195.4(B:I0) IC195.5(B:I1) IC195.6(B:O) IC195.8(C:O) IC195.9(C:I0) IC195.10(C:I1) IC195.11(D:O) IC195.12(D:I0) IC195.13(D:I1) IC196.15(G) IC197.4(B:I0) IC197.6(B:O) IC197.8(B:I1) IC197.9(B:I2) IC197.10(B:I3) IC197.11(B:I4) IC198.3(B:I) IC198.4(B:O) IC198.5(C:I) IC198.6(C:O) IC198.8(D:O) IC198.9(D:I) IC198.10(E:O) IC198.11(E:I) IC198.12(F:O) IC198.13(F:I) IC199.4(B:I0) IC199.6(B:O) IC199.8(B:I1) IC199.9(B:I2) IC199.10(B:I3) IC199.11(B:I4) IC200.1(A:I0) IC200.2(A:I1) IC200.3(A:O) IC200.8(C:O) IC200.9(C:I0) IC200.10(C:I1) IC200.11(D:O) IC200.12(D:I0) IC200.13(D:I1) IC201.1(A:I0) IC201.2(A:I1) IC201.3(A:O) IC201.4(B:I0) IC201.5(B:I1) IC201.6(B:O) IC201.11(D:O) IC201.12(D:I0) IC201.13(D:I1) IC202.11(CLK) IC203.1(A:I0) IC203.2(A:I1) IC203.3(A:O) IC203.4(B:I0) IC203.5(B:I1) IC203.6(B:O) IC203.11(D:O) IC203.12(D:I0) IC203.13(D:I1) IC204.6(A:!Q) IC204.8(B:!Q) IC204.9(B:Q) IC204.10(B:PRE) IC204.11(B:CLK) IC204.12(B:D) IC204.13(B:CLR) IC205.11(CLK) IC206.1(A:I0) IC206.2(A:I1) IC206.3(A:O) IC206.4(B:I0) IC206.5(B:I1) IC206.6(B:O) IC206.11(D:O) IC206.12(D:I0) IC206.13(D:I1) IC207.4(B:I0) IC207.5(B:I1) IC207.6(B:O) IC207.8(C:O) IC207.9(C:I0) IC207.10(C:I1) IC207.11(D:O) IC207.12(D:I0) IC207.13(D:I1) IC208.1(1G) IC208.9(2Y) IC208.10(2C0) IC208.11(2C1) IC208.12(2C2) IC208.13(2C3) IC208.15(2G) IC209.1(A:I0) IC209.2(A:I1) IC209.3(A:O) IC209.8(C:O) IC209.9(C:I0) IC209.10(C:I1) IC209.11(D:O) IC209.12(D:I0) IC209.13(D:I1) IC210.12(Y7) IC210.13(Y6) IC210.14(Y5) IC210.15(Y4) IC210.16(Y3) IC210.17(Y2) IC211.15(G) IC212.15(G) IC213.4(B:I0) IC213.5(B:I1) IC213.6(B:O) IC213.8(C:O) IC213.9(C:I0) IC213.10(C:I1) IC213.11(D:O) IC213.12(D:I0) IC213.13(D:I1) IC214.1(A:I0) IC214.2(A:I1) IC214.3(A:O) IC214.8(C:O) IC214.9(C:I0) IC214.10(C:I1) IC214.11(D:O) IC214.12(D:I0) IC214.13(D:I1) IC215.12(Y7) IC215.13(Y6) IC215.14(Y5) IC215.15(Y4) IC215.16(Y3) IC215.17(Y2) IC216.1(G) IC216.11(CLK) IC217.11(CLK) IC218.4(B:I0) IC218.5(B:I1) IC218.6(B:O) IC218.8(C:O) IC218.9(C:I0) IC218.10(C:I1) IC218.11(D:O) IC218.12(D:I0) IC218.13(D:I1) IC219.4(B:I0) IC219.5(B:I1) IC219.6(B:O) IC219.8(C:O) IC219.9(C:I0) IC219.10(C:I1) IC219.11(D:O) IC219.12(D:I0) IC219.13(D:I1) IC220.4(B:I0) IC220.5(B:I1) IC220.6(B:O) IC220.8(C:O) IC220.9(C:I0) IC220.10(C:I1) IC220.11(D:O) IC220.12(D:I0) IC220.13(D:I1) IC221.6(A:!Q) IC221.8(B:!Q) IC221.9(B:Q) IC221.10(B:PRE) IC221.11(B:CLK) IC221.12(B:D) IC221.13(B:CLR) IC223.4(B:I0) IC223.5(B:I1) IC223.6(B:O) IC223.8(C:O) IC223.9(C:I0) IC223.10(C:I1) IC223.11(D:O) IC223.12(D:I0) IC223.13(D:I1) IC224.4(B:I0) IC224.5(B:I1) IC224.6(B:O) IC224.8(C:O) IC224.9(C:I0) IC224.10(C:I1) IC224.11(D:O) IC224.12(D:I0) IC224.13(D:I1) IC225.4(B:I0) IC225.5(B:I1) IC225.6(B:O) IC225.8(C:O) IC225.9(C:I0) IC225.10(C:I1) IC225.11(D:O) IC225.12(D:I0) IC225.13(D:I1) IC227.11(CLK) IC228.1(A:I0) IC228.2(A:I1) IC228.3(A:O) IC228.4(B:I0) IC228.5(B:I1) IC228.6(B:O) IC228.11(D:O) IC228.12(D:I0) IC228.13(D:I1) IC229.4(B:I0) IC229.5(B:I1) IC229.6(B:O) IC229.8(C:O) IC229.9(C:I0) IC229.10(C:I1) IC229.11(D:O) IC229.12(D:I0) IC229.13(D:I1) IC230.1(A:I) IC230.2(A:O) IC230.5(C:I) IC230.6(C:O) IC230.8(D:O) IC230.9(D:I) IC230.10(E:O) IC230.11(E:I) IC230.12(F:O) IC230.13(F:I) IC231.1(A:I) IC231.2(A:O) IC231.4(B:O) IC231.5(C:I) IC231.6(C:O) IC231.8(D:O) IC231.9(D:I) IC231.10(E:O) IC231.11(E:I) IC231.12(F:O) IC231.13(F:I) IC232.1(A:I0) IC232.2(A:I1) IC232.3(A:O) IC232.8(C:O) IC232.9(C:I0) IC232.10(C:I1) IC232.11(D:O) IC232.12(D:I0) IC232.13(D:I1) IC233.1(A:I) IC233.2(A:O) IC233.5(C:I) IC233.6(C:O) IC233.8(D:O) IC233.9(D:I) IC233.10(E:O) IC233.11(E:I) IC233.12(F:O) IC233.13(F:I) IC235.1(A:I0) IC235.2(A:I1) IC235.3(B:I0) IC235.4(B:I1) IC235.5(B:I2) IC235.6(B:O) IC235.12(A:O) IC235.13(A:I2) IC236.1(A:I0) IC236.2(A:I1) IC236.3(B:I0) IC236.4(B:I1) IC236.5(B:I2) IC236.6(B:O) IC236.12(A:O) IC236.13(A:I2) IC237.4(B:I0) IC237.5(B:I1) IC237.6(B:O) IC237.8(C:O) IC237.9(C:I0) IC237.10(C:I1) IC237.11(D:O) IC237.12(D:I0) IC237.13(D:I1) IC238.1(A:I0) IC238.2(A:I1) IC238.3(A:O) IC238.8(C:O) IC238.9(C:I0) IC238.10(C:I1) IC238.11(D:O) IC238.12(D:I0) IC238.13(D:I1) IC241.1(1G) IC241.9(2Y) IC241.10(2C0) IC241.11(2C1) IC241.12(2C2) IC241.13(2C3) IC241.15(2G) IC242.1(A:I0) IC242.2(A:I1) IC242.3(A:O) IC242.4(B:I0) IC242.5(B:I1) IC242.6(B:O) IC242.11(D:O) IC242.12(D:I0) IC242.13(D:I1) IC243.1(1G) IC243.9(2Y) IC243.10(2C0) IC243.11(2C1) IC243.12(2C2) IC243.13(2C3) IC243.15(2G) IC244.1(A:G) IC244.2(A:A1) IC244.4(A:A2) IC244.5(B:Y3) IC244.6(A:A3) IC244.7(B:Y2) IC244.8(A:A4) IC244.12(A:Y4) IC244.14(A:Y3) IC244.16(A:Y2) IC244.18(A:Y1) IC246.11(CLK) IC247.1(A:G) IC247.2(A:A1) IC247.4(A:A2) IC247.5(B:Y3) IC247.6(A:A3) IC247.7(B:Y2) IC247.8(A:A4) IC247.12(A:Y4) IC247.14(A:Y3) IC247.16(A:Y2) IC247.18(A:Y1) IC250.1(A:I0) IC250.2(A:I1) IC250.3(A:O) IC250.8(C:O) IC250.9(C:I0) IC250.10(C:I1) IC250.11(D:O) IC250.12(D:I0) IC250.13(D:I1) IC251.11(CLK) IC252.12(Y7) IC252.13(Y6) IC252.14(Y5) IC252.15(Y4) IC252.16(Y3) IC252.17(Y2) IC253.12(Y7) IC253.13(Y6) IC253.14(Y5) IC253.15(Y4) IC253.16(Y3) IC253.17(Y2) IC254.11(CLK) IC255.1(1G) IC255.9(2Y) IC255.10(2C0) IC255.11(2C1) IC255.12(2C2) IC255.13(2C3) IC255.15(2G) IC256.1(1G) IC256.9(2Y) IC256.10(2C0) IC256.11(2C1) IC256.12(2C2) IC256.13(2C3) IC256.15(2G) IC257.15(G) IC259.12(Y7) IC259.13(Y6) IC259.14(Y5) IC259.15(Y4) IC259.16(Y3) IC259.17(Y2) IC260.12(Y7) IC260.13(Y6) IC260.14(Y5) IC260.15(Y4) IC260.16(Y3) IC260.17(Y2) IC261.11(CLK) IC262.11(CLK) IC263.12(Y7) IC263.13(Y6) IC263.14(Y5) IC263.15(Y4) IC263.16(Y3) IC263.17(Y2) IC264.12(Y7) IC264.13(Y6) IC264.14(Y5) IC264.15(Y4) IC264.16(Y3) IC264.17(Y2) IC265.11(CLK) IC266.12(Y7) IC266.13(Y6) IC266.14(Y5) IC266.15(Y4) IC266.16(Y3) IC266.17(Y2) IC267.12(Y7) IC267.13(Y6) IC267.14(Y5) IC267.15(Y4) IC267.16(Y3) IC267.17(Y2) IC269.4(B:I0) IC269.5(B:I1) IC269.6(B:O) IC269.8(C:O) IC269.9(C:I0) IC269.10(C:I1) IC269.11(D:O) IC269.12(D:I0) IC269.13(D:I1) IC270.1(A:I) IC270.2(A:O) IC270.5(C:I) IC270.6(C:O) IC270.8(D:O) IC270.9(D:I) IC270.10(E:O) IC270.11(E:I) IC270.12(F:O) IC270.13(F:I) IC271.1(A:I) IC271.2(A:O) IC271.5(C:I) IC271.6(C:O) IC271.8(D:O) IC271.9(D:I) IC271.10(E:O) IC271.11(E:I) IC271.12(F:O) IC271.13(F:I) IC272.1(!A!/B) IC277.1(!A!/B) IC287.9(C4) IC288.3(B:Y4) IC288.5(B:Y3) IC288.7(B:Y2) IC288.9(B:Y1) IC288.11(B:A1) IC288.13(B:A2) IC288.15(B:A3) IC288.17(B:A4) IC288.19(B:G) IC289.3(B:Y4) IC289.5(B:Y3) IC289.7(B:Y2) IC289.9(B:Y1) IC289.11(B:A1) IC289.13(B:A2) IC289.15(B:A3) IC289.17(B:A4) IC289.19(B:G) IC290.3(B:Y4) IC290.5(B:Y3) IC290.7(B:Y2) IC290.9(B:Y1) IC290.11(B:A1) IC290.13(B:A2) IC290.15(B:A3) IC290.17(B:A4) IC290.19(B:G) IC291.3(B:Y4) IC291.5(B:Y3) IC291.7(B:Y2) IC291.9(B:Y1) IC291.11(B:A1) IC291.13(B:A2) IC291.15(B:A3) IC291.17(B:A4) IC291.19(B:G) IC292.3(B:Y4) IC292.5(B:Y3) IC292.7(B:Y2) IC292.9(B:Y1) IC292.11(B:A1) IC292.13(B:A2) IC292.15(B:A3) IC292.17(B:A4) IC292.19(B:G) IC293.3(B:Y4) IC293.5(B:Y3) IC293.7(B:Y2) IC293.9(B:Y1) IC293.11(B:A1) IC293.13(B:A2) IC293.15(B:A3) IC293.17(B:A4) IC293.19(B:G) IC294.3(B:Y4) IC294.5(B:Y3) IC294.7(B:Y2) IC294.9(B:Y1) IC294.11(B:A1) IC294.13(B:A2) IC294.15(B:A3) IC294.17(B:A4) IC294.19(B:G) IC295.3(B:Y4) IC295.5(B:Y3) IC295.7(B:Y2) IC295.9(B:Y1) IC295.11(B:A1) IC295.13(B:A2) IC295.15(B:A3) IC295.17(B:A4) IC295.19(B:G) IC296.11(CLK) IC297.3(B:Y4) IC297.5(B:Y3) IC297.7(B:Y2) IC297.9(B:Y1) IC297.11(B:A1) IC297.13(B:A2) IC297.15(B:A3) IC297.17(B:A4) IC297.19(B:G) IC298.3(B:Y4) IC298.5(B:Y3) IC298.7(B:Y2) IC298.9(B:Y1) IC298.11(B:A1) IC298.13(B:A2) IC298.15(B:A3) IC298.17(B:A4) IC298.19(B:G) IC299.3(B:Y4) IC299.5(B:Y3) IC299.7(B:Y2) IC299.9(B:Y1) IC299.11(B:A1) IC299.13(B:A2) IC299.15(B:A3) IC299.17(B:A4) IC299.19(B:G) IC300.3(B:Y4) IC300.5(B:Y3) IC300.7(B:Y2) IC300.9(B:Y1) IC300.11(B:A1) IC300.13(B:A2) IC300.15(B:A3) IC300.17(B:A4) IC300.19(B:G) IC301.11(CLK) IC302.12(Y7) IC302.13(Y6) IC302.14(Y5) IC302.15(Y4) IC302.16(Y3) IC302.17(Y2) IC303.12(Y7) IC303.13(Y6) IC303.14(Y5) IC303.15(Y4) IC303.16(Y3) IC303.17(Y2) IC410.1(A:I) IC410.2(A:O) IC410.5(C:I) IC410.6(C:O) IC410.8(D:O) IC410.9(D:I) IC410.10(E:O) IC410.11(E:I) IC410.12(F:O) IC410.13(F:I) IC411.2(A:S1) IC411.5(C:R) IC411.6(C:S) IC411.7(C:Q) IC411.9(B:Q) IC411.10(B:R) IC411.11(B:S1) IC411.12(B:S2) IC411.13(D:Q) IC411.14(D:R) IC411.15(D:S) IC412.4(Q2) IC412.5(Q3) IC412.6(Q4) IC412.11(D4) IC412.12(D3) IC412.13(D2) IC413.6(A:!Q) IC413.8(B:!Q) IC413.9(B:Q) IC413.10(B:PRE) IC413.11(B:CLK) IC413.12(B:D) IC413.13(B:CLR) IC414.1(A:I) IC414.2(A:O) IC414.5(C:I) IC414.6(C:O) IC414.8(D:O) IC414.9(D:I) IC414.10(E:O) IC414.11(E:I) IC414.12(F:O) IC414.13(F:I) IC415.1(A:I0) IC415.2(A:I1) IC415.3(A:O) IC415.8(C:O) IC415.9(C:I0) IC415.10(C:I1) IC415.11(D:O) IC415.12(D:I0) IC415.13(D:I1) IC544.11(CLK) RN4.4 RN4.5 RN4.6 RN4.7 RN4.8 RN4.9 RN4.10 RN4.11 RN4.12 RN4.13 S5.1(O) S6.1(O) SW1.8 U$1.28(VCC) U$2.28(VCC) U$3.28(VCC) U$4.28(VCC) U$5.28(VCC) U$6.28(VCC) U$7.28(VCC) U$8.28(VCC) U$9.28(VCC) U$10.1(A14) U$10.2(A12) U$10.3(A7) U$10.4(A6) U$10.5(A5) U$10.6(A4) U$10.7(A3) U$10.8(A2) U$10.9(A1) U$10.10(A0) U$10.14(GND) U$10.20(/CE) U$10.21(A10) U$10.22(/OE) U$10.23(A11) U$10.24(A9) U$10.25(A8) U$10.26(A13) U$10.27(/WE) U$10.28(VCC) U$11.1(A14) U$11.2(A12) U$11.3(A7) U$11.4(A6) U$11.5(A5) U$11.6(A4) U$11.7(A3) U$11.8(A2) U$11.9(A1) U$11.10(A0) U$11.14(GND) U$11.20(/CE) U$11.21(A10) U$11.22(/OE) U$11.23(A11) U$11.24(A9) U$11.25(A8) U$11.26(A13) U$11.27(/WE) U$11.28(VCC) U$12.1(A14) U$12.2(A12) U$12.3(A7) U$12.4(A6) U$12.5(A5) U$12.6(A4) U$12.7(A3) U$12.8(A2) U$12.9(A1) U$12.10(A0) U$12.14(GND) U$12.20(/CE) U$12.21(A10) U$12.22(/OE) U$12.23(A11) U$12.24(A9) U$12.25(A8) U$12.26(A13) U$12.27(/WE) U$12.28(VCC)

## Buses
XBUS[0..7]
ZBUS[0..7]
YBUS[0..7]
AD[0..19]
MDR_IN_BUS[0..7]
U_AD[0..15]
DATA[0..7]

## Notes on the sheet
- The codename DreamCatcher homemade 8/16bit CPU/Minicomputer
  Conceived & designed by Paulo Constantino - pconst167@gmail.com
  
  The purpose of designing this CPU/Minicomputer was manyfold. 
  Firstly it will be aimed at students who are looking for practice in 
  building computer CPU's and systems. 
  Seconly, it will be connected to the internet by myself (and maybe others who will follow) 
  and used to host a bulletin-board like system whereby enthusiasts and students can log-on, 
  download files, schematics, use forums, chat, play games, and many other activities. 
  This should inspire people to study and build it, if they see that it works well. 
  And lastly, designing and building computers is just pure ecstasy!!
  
  Shareware - Share with passion!!
  
  This file is probably a .png image. For the original Eagle schematics, ask by e-mail!
- DMA CAN ONLY HAPPEN IF WE ARE NOT TRAPPING.
- SYNCHRONIZED INTERRUPT INPUTS
- INT_REQ_0
  INT_REQ_1
  INT_REQ_2
  INT_REQ_3
  INT_REQ_4
  INT_REQ_5
  INT_REQ_6
  INT_REQ_7
- SINGLE STEP CLOCK
- thevenin termination at the far end of the Z bus. (not ALU's end)
- IF A TRAP HAPPENS, THEN NEITHER MASKABLE INTERRUPTS
  NOR TRAPS ARE ALLOWED TO HAPPEN.
  
  THIS IS DICTATED BY THE TRAP_ENABLE SIGNAL
- IMMX
- the encoded bits start at position 3 in the byte. 
  this is so it's easier to just transfer this to PC and 
  have it become the interrupt vector in memory.
  
  so each interrupt spans 8 bytes in memory.
  
  00000000 = int_0
  00001000 = int_1
  00010000 = int_2
  00011000 = int_3
  etc
- R_SHIFT_L
- U-ADDRESS MUX
- R_SHIFT_H
- CS_L
- MASK_FLAGS
- CS_H
- ADDRESS & DATA BUSES NEED PULL DOWN RESISTORS 
  BECAUSE THE CPU BUS OUTPUTS HAVE 
  244'S WHICH ARE CLOSED MOST OF THE TIME.
- LOW
- DS_L
- OFFSET(6)
- DS_H
- IR_L
- AL
- Z BUS
- PC_L
- SS_L
- AH
- U-CODE ROMS
- U-ADDRESS
- U-CODE FF'S
- MARL
- SS_H
- IR_H
- PC_H
- BL
- LOW
- LOW | ES_L
- ADDER | HIGH
- HIGH
- BH
- MARH
- MAR is tri-stated when in programming or DMA mode.
- ES_H
- programming mode signal goes here to tell MAR to go tristate
- AUX_FLAGS
- CL | SP_L
- ADDER
- upper bits are a copy of u_offset6. this means this offset
  is a signed number from -64 to 63
- SI_L
- CH
- SP_H
- SI_H
- if type = branch, and condition = false, then next = +1
- DL | BP_L
- HIGH
- Z BUS
- DI_L
- DH | BP_H
- FLAGS REGISTER
- DI_H
- CARRY IN MUX
- U_FLAGS
- BUS GOING INTO MDR INPUTS
- MDRL_L
- DATA BUS
- CONDITION SOURCE
  PROGRAMMER'S FLAGS 
  OR
  U_CODE FLAGS
- MDRL_H
- ZF | MDR MUX | BUS GOING INTO MDR INPUTS
- CF / LTU
- SF
- IMMY
- OF
- ALU
- PF | TDR_L
- alu_mode removed. OF is undefined if alu in logic mode anyway. | alu_op == add
- LT
  LTE
  ~LT = GTE
  ~LTE + GT
- TDR_H
- DATA BUS
- SERIES TERMINATION ~80 ohm
- ALU_OP == SUB
- IMMY
- FROM MICROCODE
- MDRH_L
- MDRH_H
- DATA BUS

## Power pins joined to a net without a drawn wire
GND: IC1.10(GND) IC2.10(GND) IC3.10(GND) IC4.10(GND) IC5.10(GND) IC6.10(GND) IC7.10(GND) IC8.7(P:GND) IC9.10(GND) IC10.10(P:GND) IC11.10(P:GND) IC12.10(P:GND) IC13.10(P:GND) IC14.12(GND) IC15.12(GND) IC16.10(GND) IC17.10(GND) IC18.7(P:GND) IC19.10(GND) IC20.8(GND) IC21.10(GND) IC22.8(GND) IC23.8(GND) IC24.10(P:GND) IC25.10(P:GND) IC26.10(P:GND) IC27.10(P:GND) IC28.10(GND) IC29.10(GND) IC30.10(P:GND) IC31.10(P:GND) IC32.10(GND) IC33.10(GND) IC34.8(GND) IC35.8(GND) IC36.8(GND) IC37.8(GND) IC38.8(GND) IC39.7(P:GND) IC40.8(GND) IC41.8(GND) IC42.7(P:GND) IC43.7(P:GND) IC44.10(GND) IC45.7(P:GND) IC46.7(P:GND) IC47.7(P:GND) IC48.10(GND) IC49.8(GND) IC50.8(GND) IC51.8(GND) IC52.8(GND) IC53.8(GND) IC54.10(GND) IC55.8(GND) IC56.8(GND) IC57.7(P:GND) IC58.7(P:GND) IC59.7(P:GND) IC60.10(GND) IC61.10(GND) IC62.10(GND) IC63.8(GND) IC64.7(P:GND) IC65.7(P:GND) IC66.7(P:GND) IC68.8(GND) IC69.10(P:GND) IC70.8(GND) IC71.8(GND) IC72.7(P:GND) IC73.8(GND) IC74.7(P:GND) IC75.10(GND) IC76.10(GND) IC77.10(GND) IC78.10(GND) IC79.10(GND) IC80.7(P:GND) IC81.7(P:GND) IC82.7(P:GND) IC83.7(P:GND) IC84.7(P:GND) IC85.7(P:GND) IC86.8(GND) IC87.10(GND) IC88.8(GND) IC89.8(GND) IC90.8(GND) IC91.10(GND) IC92.10(GND) IC93.7(P:GND) IC94.7(P:GND) IC95.8(GND) IC96.8(GND) IC97.8(GND) IC98.10(GND) IC99.10(GND) IC100.10(GND) IC101.10(GND) IC102.10(GND) IC103.8(GND) IC104.8(GND) IC105.10(P:GND) IC106.10(P:GND) IC107.10(P:GND) IC108.10(P:GND) IC109.10(P:GND) IC110.10(P:GND) IC111.10(P:GND) IC112.10(P:GND) IC113.10(GND) IC114.10(GND) IC115.10(GND) IC116.10(GND) IC117.10(GND) IC118.10(GND) IC119.8(GND) IC120.7(P:GND) IC121.8(GND) IC122.10(GND) IC123.10(GND) IC124.8(GND) IC125.10(GND) IC126.10(GND) IC127.7(P:GND) IC128.8(GND) IC129.8(GND) IC130.7(P:GND) IC131.7(P:GND) IC132.7(P:GND) IC133.7(P:GND) IC134.10(GND) IC135.10(GND) IC136.10(GND) IC137.10(GND) IC138.7(P:GND) IC139.10(GND) IC140.10(GND) IC141.7(P:GND) IC142.8(GND) IC143.7(P:GND) IC144.8(GND) IC145.10(GND) IC146.10(GND) IC147.7(P:GND) IC148.8(GND) IC149.7(P:GND) IC150.7(P:GND) IC151.7(P:GND) IC152.7(P:GND) IC153.10(GND) IC154.10(GND) IC155.8(GND) IC156.8(GND) IC157.7(P:GND) IC158.7(P:GND) IC159.8(GND) IC160.8(GND) IC161.8(GND) IC162.10(GND) IC163.7(P:GND) IC164.7(P:GND) IC165.10(GND) IC166.10(GND) IC167.8(GND) IC168.7(P:GND) IC169.10(GND) IC170.7(P:GND) IC171.10(GND) IC172.8(GND) IC173.10(GND) IC174.7(P:GND) IC175.7(P:GND) IC176.10(P:GND) IC177.7(P:GND) IC178.10(P:GND) IC179.10(P:GND) IC180.10(GND) IC181.10(P:GND) IC182.10(P:GND) IC183.10(P:GND) IC184.10(GND) IC185.10(GND) IC186.8(GND) IC187.7(P:GND) IC188.7(P:GND) IC189.10(GND) IC190.7(P:GND) IC191.7(P:GND) IC192.7(P:GND) IC193.7(P:GND) IC194.7(P:GND) IC195.7(P:GND) IC196.8(GND) IC197.7(P:GND) IC198.7(P:GND) IC199.7(P:GND) IC200.7(P:GND) IC201.7(P:GND) IC202.10(GND) IC203.7(P:GND) IC204.7(P:GND) IC205.10(GND) IC206.7(P:GND) IC207.7(P:GND) IC208.8(GND) IC209.7(P:GND) IC210.10(GND) IC211.8(GND) IC212.8(GND) IC213.7(P:GND) IC214.7(P:GND) IC215.10(GND) IC216.10(GND) IC217.10(GND) IC218.7(P:GND) IC219.7(P:GND) IC220.7(P:GND) IC221.7(P:GND) IC222.8(GND) IC223.7(P:GND) IC224.7(P:GND) IC225.7(P:GND) IC226.8(GND) IC227.10(GND) IC228.7(P:GND) IC229.7(P:GND) IC230.7(P:GND) IC231.7(P:GND) IC232.7(P:GND) IC233.7(P:GND) IC235.7(P:GND) IC236.7(P:GND) IC237.7(P:GND) IC238.7(P:GND) IC241.8(GND) IC242.7(P:GND) IC243.8(GND) IC244.10(P:GND) IC245.10(GND) IC246.10(GND) IC247.10(P:GND) IC248.8(GND) IC249.8(GND) IC250.7(P:GND) IC251.10(GND) IC252.10(GND) IC253.10(GND) IC254.10(GND) IC255.8(GND) IC256.8(GND) IC257.8(GND) IC258.8(GND) IC259.10(GND) IC260.10(GND) IC261.10(GND) IC262.10(GND) IC263.10(GND) IC264.10(GND) IC265.10(GND) IC266.10(GND) IC267.10(GND) IC268.8(GND) IC269.7(P:GND) IC270.7(P:GND) IC271.7(P:GND) IC272.8(GND) IC273.8(GND) IC274.8(GND) IC275.8(GND) IC276.8(GND) IC277.8(GND) IC278.8(GND) IC279.8(GND) IC280.8(GND) IC281.8(GND) IC282.8(GND) IC283.8(GND) IC284.8(GND) IC285.8(GND) IC286.8(GND) IC287.8(GND) IC288.10(P:GND) IC289.10(P:GND) IC290.10(P:GND) IC291.10(P:GND) IC292.10(P:GND) IC293.10(P:GND) IC294.10(P:GND) IC295.10(P:GND) IC296.10(GND) IC297.10(P:GND) IC298.10(P:GND) IC299.10(P:GND) IC300.10(P:GND) IC301.10(GND) IC302.10(GND) IC303.10(GND) IC410.7(P:GND) IC411.8(P:GND) IC412.8(GND) IC413.7(P:GND) IC414.7(P:GND) IC415.7(P:GND) IC544.10(GND)
VCC: IC1.20(VCC) IC2.20(VCC) IC3.20(VCC) IC4.20(VCC) IC5.20(VCC) IC6.20(VCC) IC7.20(VCC) IC8.14(P:VCC) IC9.20(VCC) IC10.20(P:VCC) IC11.20(P:VCC) IC12.20(P:VCC) IC13.20(P:VCC) IC14.24(VCC) IC15.24(VCC) IC16.20(VCC) IC17.20(VCC) IC18.14(P:VCC) IC19.20(VCC) IC20.16(VCC) IC21.20(VCC) IC22.16(VCC) IC23.16(VCC) IC24.20(P:VCC) IC25.20(P:VCC) IC26.20(P:VCC) IC27.20(P:VCC) IC28.20(VCC) IC29.20(VCC) IC30.20(P:VCC) IC31.20(P:VCC) IC32.20(VCC) IC33.20(VCC) IC34.16(VCC) IC35.16(VCC) IC36.16(VCC) IC37.16(VCC) IC38.16(VCC) IC39.14(P:VCC) IC40.16(VCC) IC41.16(VCC) IC42.14(P:VCC) IC43.14(P:VCC) IC44.20(VCC) IC45.14(P:VCC) IC46.14(P:VCC) IC47.14(P:VCC) IC48.20(VCC) IC49.16(VCC) IC50.16(VCC) IC51.16(VCC) IC52.16(VCC) IC53.16(VCC) IC54.20(VCC) IC55.16(VCC) IC56.16(VCC) IC57.14(P:VCC) IC58.14(P:VCC) IC59.14(P:VCC) IC60.20(VCC) IC61.20(VCC) IC62.20(VCC) IC63.16(VCC) IC64.14(P:VCC) IC65.14(P:VCC) IC66.14(P:VCC) IC68.16(VCC) IC69.20(P:VCC) IC70.16(VCC) IC71.16(VCC) IC72.14(P:VCC) IC73.16(VCC) IC74.14(P:VCC) IC75.20(VCC) IC76.20(VCC) IC77.20(VCC) IC78.20(VCC) IC79.20(VCC) IC80.14(P:VCC) IC81.14(P:VCC) IC82.14(P:VCC) IC83.14(P:VCC) IC84.14(P:VCC) IC85.14(P:VCC) IC86.16(VCC) IC87.20(VCC) IC88.16(VCC) IC89.16(VCC) IC90.16(VCC) IC91.20(VCC) IC92.20(VCC) IC93.14(P:VCC) IC94.14(P:VCC) IC95.16(VCC) IC96.16(VCC) IC97.16(VCC) IC98.20(VCC) IC99.20(VCC) IC100.20(VCC) IC101.20(VCC) IC102.20(VCC) IC103.16(VCC) IC104.16(VCC) IC105.20(P:VCC) IC106.20(P:VCC) IC107.20(P:VCC) IC108.20(P:VCC) IC109.20(P:VCC) IC110.20(P:VCC) IC111.20(P:VCC) IC112.20(P:VCC) IC113.20(VCC) IC114.20(VCC) IC115.20(VCC) IC116.20(VCC) IC117.20(VCC) IC118.20(VCC) IC119.16(VCC) IC120.14(P:VCC) IC121.16(VCC) IC122.20(VCC) IC123.20(VCC) IC124.16(VCC) IC125.20(VCC) IC126.20(VCC) IC127.14(P:VCC) IC128.16(VCC) IC129.16(VCC) IC130.14(P:VCC) IC131.14(P:VCC) IC132.14(P:VCC) IC133.14(P:VCC) IC134.20(VCC) IC135.20(VCC) IC136.20(VCC) IC137.20(VCC) IC138.14(P:VCC) IC139.20(VCC) IC140.20(VCC) IC141.14(P:VCC) IC142.16(VCC) IC143.14(P:VCC) IC144.16(VCC) IC145.20(VCC) IC146.20(VCC) IC147.14(P:VCC) IC148.16(VCC) IC149.14(P:VCC) IC150.14(P:VCC) IC151.14(P:VCC) IC152.14(P:VCC) IC153.20(VCC) IC154.20(VCC) IC155.16(VCC) IC156.16(VCC) IC157.14(P:VCC) IC158.14(P:VCC) IC159.16(VCC) IC160.16(VCC) IC161.16(VCC) IC162.20(VCC) IC163.14(P:VCC) IC164.14(P:VCC) IC165.20(VCC) IC166.20(VCC) IC167.16(VCC) IC168.14(P:VCC) IC169.20(VCC) IC170.14(P:VCC) IC171.20(VCC) IC172.16(VCC) IC173.20(VCC) IC174.14(P:VCC) IC175.14(P:VCC) IC176.20(P:VCC) IC177.14(P:VCC) IC178.20(P:VCC) IC179.20(P:VCC) IC180.20(VCC) IC181.20(P:VCC) IC182.20(P:VCC) IC183.20(P:VCC) IC184.20(VCC) IC185.20(VCC) IC186.16(VCC) IC187.14(P:VCC) IC188.14(P:VCC) IC189.20(VCC) IC190.14(P:VCC) IC191.14(P:VCC) IC192.14(P:VCC) IC193.14(P:VCC) IC194.14(P:VCC) IC195.14(P:VCC) IC196.16(VCC) IC197.14(P:VCC) IC198.14(P:VCC) IC199.14(P:VCC) IC200.14(P:VCC) IC201.14(P:VCC) IC202.20(VCC) IC203.14(P:VCC) IC204.14(P:VCC) IC205.20(VCC) IC206.14(P:VCC) IC207.14(P:VCC) IC208.16(VCC) IC209.14(P:VCC) IC210.20(VCC) IC211.16(VCC) IC212.16(VCC) IC213.14(P:VCC) IC214.14(P:VCC) IC215.20(VCC) IC216.20(VCC) IC217.20(VCC) IC218.14(P:VCC) IC219.14(P:VCC) IC220.14(P:VCC) IC221.14(P:VCC) IC222.16(VCC) IC223.14(P:VCC) IC224.14(P:VCC) IC225.14(P:VCC) IC226.16(VCC) IC227.20(VCC) IC228.14(P:VCC) IC229.14(P:VCC) IC230.14(P:VCC) IC231.14(P:VCC) IC232.14(P:VCC) IC233.14(P:VCC) IC235.14(P:VCC) IC236.14(P:VCC) IC237.14(P:VCC) IC238.14(P:VCC) IC241.16(VCC) IC242.14(P:VCC) IC243.16(VCC) IC244.20(P:VCC) IC245.20(VCC) IC246.20(VCC) IC247.20(P:VCC) IC248.16(VCC) IC249.16(VCC) IC250.14(P:VCC) IC251.20(VCC) IC252.20(VCC) IC253.20(VCC) IC254.20(VCC) IC255.16(VCC) IC256.16(VCC) IC257.16(VCC) IC258.16(VCC) IC259.20(VCC) IC260.20(VCC) IC261.20(VCC) IC262.20(VCC) IC263.20(VCC) IC264.20(VCC) IC265.20(VCC) IC266.20(VCC) IC267.20(VCC) IC268.16(VCC) IC269.14(P:VCC) IC270.14(P:VCC) IC271.14(P:VCC) IC272.16(VCC) IC273.16(VCC) IC274.16(VCC) IC275.16(VCC) IC276.16(VCC) IC277.16(VCC) IC278.16(VCC) IC279.16(VCC) IC280.16(VCC) IC281.16(VCC) IC282.16(VCC) IC283.16(VCC) IC284.16(VCC) IC285.16(VCC) IC286.16(VCC) IC287.16(VCC) IC288.20(P:VCC) IC289.20(P:VCC) IC290.20(P:VCC) IC291.20(P:VCC) IC292.20(P:VCC) IC293.20(P:VCC) IC294.20(P:VCC) IC295.20(P:VCC) IC296.20(VCC) IC297.20(P:VCC) IC298.20(P:VCC) IC299.20(P:VCC) IC300.20(P:VCC) IC301.20(VCC) IC302.20(VCC) IC303.20(VCC) IC410.14(P:VCC) IC411.16(P:VCC) IC412.16(VCC) IC413.14(P:VCC) IC414.14(P:VCC) IC415.14(P:VCC) IC544.20(VCC)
